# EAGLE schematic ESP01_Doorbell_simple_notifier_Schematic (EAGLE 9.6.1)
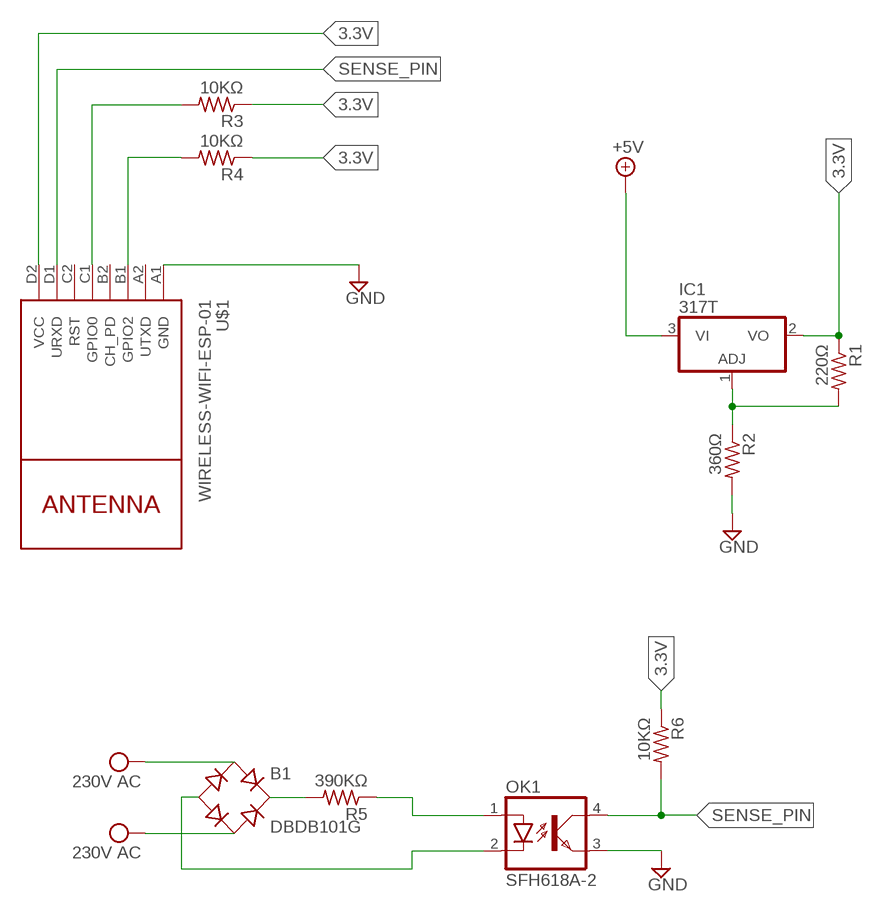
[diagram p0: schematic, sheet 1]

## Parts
B1  DBDB101G  [DB]
IC1  317T  [TO220H]
OK1  SFH618A-2  [DIP4]
R1  220Ω  R-US_0204/5  [0204/5]
R2  360Ω  R-US_0204/5  [0204/5]
R3  10KΩ  R-US_0204/5  [0204/5]
R4  10KΩ  R-US_0204/5  [0204/5]
R5  390KΩ  R-US_0204/5  [0204/5]
R6  10KΩ  R-US_0204/5  [0204/5]
U$1  WIRELESS-WIFI-ESP-01  [WIRELESS-WIFI-ESP-01]

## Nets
3.3V: IC1.2(VO) R1.1 R3.1 R4.1 U$1.D2(VCC)
+5V: IC1.3(VI)
GND: OK1.3(EMIT) R2.2 U$1.A1(GND)
N$1: R4.2 U$1.B1(GPIO2)
N$2: IC1.1(ADJ) R1.2 R2.1
N$3: R3.2 U$1.C1(GPIO0)
N$4: B1.- OK1.2(C)
N$5: B1.+ R5.2
N$6: OK1.1(A) R5.1
N$7: OK1.4(COL) R6.2
N$8: R6.1
SENSE_PIN: U$1.D1(URXD)
VCC: B1.AC1 B1.AC2 ; supply symbol labelled 230V AC
Unconnected: U$1.A2(UTXD) U$1.B2(CH_PD) U$1.C2(RST)

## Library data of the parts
B1 = rectifier:DB?*G: Single Phase 1.0 AMP Glass Passivated Bridge Rectifier Taiwan Semiconductor Co.,Ltd. - TSC Source: http://www.taiwansemi.com/TSCbig5/ezcatfiles/cust/img/img/db101g.pdf http://www.ts.com.tw/db/pictures/modules/PDT/PDT060207001/DBLS201G.pdf
IC1 = linear:*317: Positive VOLTAGE REGULATOR
OK1 = optocoupler:SFH618?*: Optocoupler, Phototransistor Output, Low Input Current Source: Data sheet; MF: VISHAY/TELEFUNKEN; MPN: SFH618A-2; OC_FARNELL: 6424855; OC_NEWARK: 21H7744
R1-R6 = resistor:R-US_: RESISTOR, American symbol
U$1 = diy-modules:WIRELESS-WIFI-ESP-01: Wireless Wi-Fi ESP-01 Module based on ESP8266 chip Click here to find device on ebay.com

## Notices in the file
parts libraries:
diy-modules: Released under the Creative Commons Attribution 4.0 International License: http://creativecommons.org/licenses/by/4.0
